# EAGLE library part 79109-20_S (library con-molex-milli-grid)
RECEPTACAL
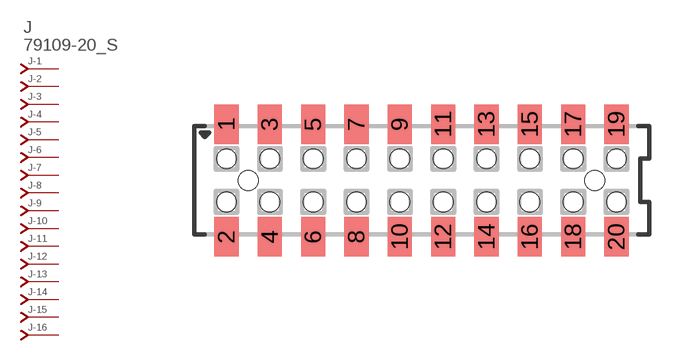
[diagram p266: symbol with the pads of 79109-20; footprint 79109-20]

Designator prefix J; gates -1=J-NV -2=J-N -3=J-N -4=J-N -5=J-N -6=J-N -7=J-N -8=J-N -9=J-N -10=J-N -11=J-N -12=J-N -13=J-N -14=J-N -15=J-N -16=J-N -17=J-N -18=J-N -19=J-N -20=J-N

## 79109-20_S  [79109-20]
1  -1:J  pas
2  -2:J  pas
3  -3:J  pas
4  -4:J  pas
5  -5:J  pas
6  -6:J  pas
7  -7:J  pas
8  -8:J  pas
9  -9:J  pas
10  -10:J  pas
11  -11:J  pas
12  -12:J  pas
13  -13:J  pas
14  -14:J  pas
15  -15:J  pas
16  -16:J  pas
17  -17:J  pas
18  -18:J  pas
19  -19:J  pas
20  -20:J  pas

## Footprint 79109-20 (pad centres in mm)
RECEPTACAL SMD Dual Row, Vertical, Pass-Thru
smd 1.12 x 1.83: 1 -9,2.6; 2 -9,-2.6; 3 -7,2.6; 4 -7,-2.6; 5 -5,2.6; 6 -5,-2.6; 7 -3,2.6; 8 -3,-2.6; 9 -1,2.6; 10 -1,-2.6; 11 1,2.6; 12 1,-2.6; 13 3,2.6; 14 3,-2.6; 15 5,2.6; 16 5,-2.6; 17 7,2.6; 18 7,-2.6; 19 9,2.6; 20 9,-2.6
hole 0.914 at -8,0
hole 0.914 at -9,1
hole 0.914 at -9,-1
hole 0.914 at -7,-1
hole 0.914 at -7,1
hole 0.914 at -5,-1
hole 0.914 at -5,1
hole 0.914 at 8,0
hole 0.914 at -3,1
hole 0.914 at -3,-1
hole 0.914 at -1,1
hole 0.914 at -1,-1
hole 0.914 at 1,1
hole 0.914 at 1,-1
hole 0.914 at 3,1
hole 0.914 at 3,-1
hole 0.914 at 5,-1
hole 0.914 at 5,1
hole 0.914 at 7,1
hole 0.914 at 7,-1
hole 0.914 at 9,1
hole 0.914 at 9,-1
